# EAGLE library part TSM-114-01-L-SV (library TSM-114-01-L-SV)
Headers & Wire Housings .100" Surface Mount Terminal Strip Source: Datasheet
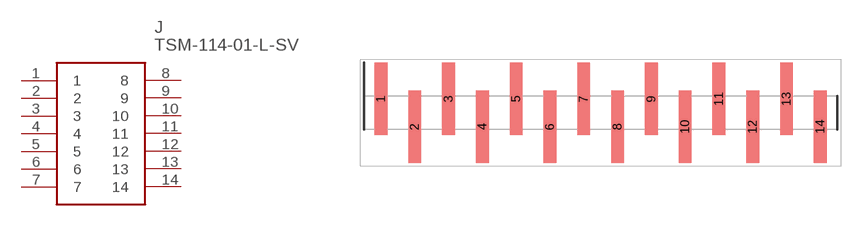
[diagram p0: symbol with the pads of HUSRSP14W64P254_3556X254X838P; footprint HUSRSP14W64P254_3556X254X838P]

Designator prefix J

## TSM-114-01-L-SV (Description: Headers & Wire Housings .100" Surface Mount Terminal Strip; Height: mm; Manufacturer_Name: SAMTEC; Manufacturer_Part_Number: TSM-114-01-L-SV; Mouser_Part_Number: 200-TSM11401LSV; Mouser_Price-Stock: https://www.mouser.com/Search/Refine.aspx?Keyword=200-TSM11401LSV)  [HUSRSP14W64P254_3556X254X838P]
1  1
2  2
3  3
4  4
5  5
6  6
7  7
8  8
9  9
10  10
11  11
12  12
13  13
14  14

## Footprint HUSRSP14W64P254_3556X254X838P (pad centres in mm)
TSM-114-01-L-SV-
smd 0.96 x 5.46: 1 -16.51,1.045; 2 -13.97,-1.045; 3 -11.43,1.045; 4 -8.89,-1.045; 5 -6.35,1.045; 6 -3.81,-1.045; 7 -1.27,1.045; 8 1.27,-1.045; 9 3.81,1.045; 10 6.35,-1.045; 11 8.89,1.045; 12 11.43,-1.045; 13 13.97,1.045; 14 16.51,-1.045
